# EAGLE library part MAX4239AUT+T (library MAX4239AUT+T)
MAXIM INTEGRATED PRODUCTS - MAX4239AUT+T - OP AMP, 6.5MHZ, 1.6V/US, SOT23-6 Source: Datasheet
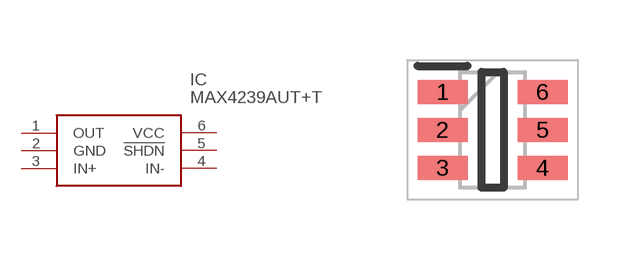
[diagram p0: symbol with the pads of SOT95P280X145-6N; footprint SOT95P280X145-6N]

Designator prefix IC

## MAX4239AUT+T (Description: MAXIM INTEGRATED PRODUCTS - MAX4239AUT+T - OP AMP, 6.5MHZ, 1.6V/US, SOT23-6; Height: 1.45mm; Manufacturer_Name: Analog Devices; Manufacturer_Part_Number: MAX4239AUT+T; Mouser_Part_Number: 700-MAX4239AUT+T; Mouser_Price-Stock: https://www.mouser.co.uk/ProductDetail/Analog-Devices-Maxim-Integrated/MAX4239AUT%2bT?qs=Mc2rGIXtnyWh0Jhb9STGCw%3D%3D)  [SOT95P280X145-6N]
1  OUT
2  GND
3  IN+
4  IN-
5  !SHDN
6  VCC

## Footprint SOT95P280X145-6N (pad centres in mm)
21-0058
smd 1.25 x 0.6: 1 -1.25,0.95; 2 -1.25,0; 3 -1.25,-0.95; 4 1.25,-0.95; 5 1.25,0; 6 1.25,0.95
